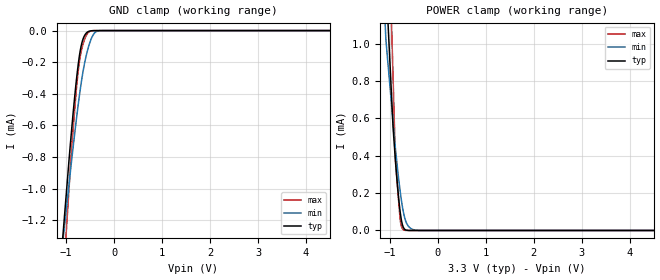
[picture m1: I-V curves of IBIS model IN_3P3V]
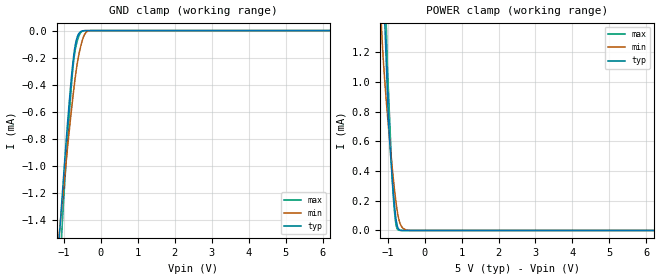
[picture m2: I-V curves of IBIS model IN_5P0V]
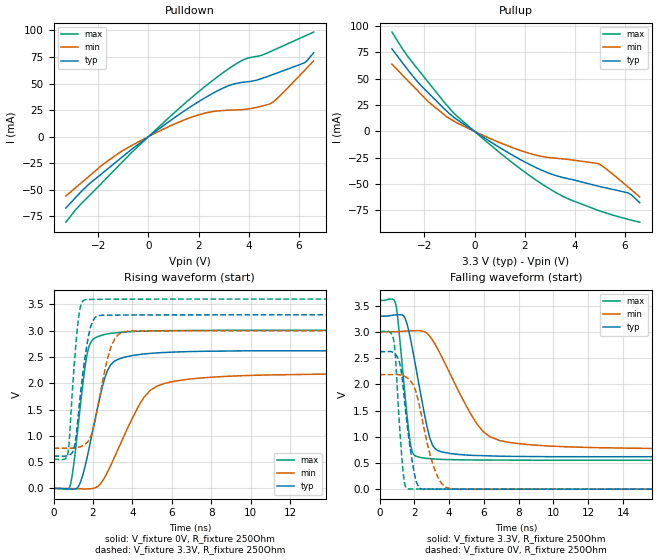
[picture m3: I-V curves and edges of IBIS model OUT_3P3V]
| Texas Instruments Incorporated
| Low-Power Single channel Digital Isolator
| Marketing part#   Voltage Range   Package-type   #pins/pkg drawing
| ISO7310C   3.0V - 5.5V   SOIC   8-pin D
[IBIS Ver]   4.1
[File name]   iso7310fc.ibs
[File Rev]   1.0
[Date]   09/30/2014
[Source]   Model built from spectre simulations at:
   Texas Instruments Incorporated.
   Analog-eLab, HPA
   12500 TI Blvd
   Dallas, TX -75243
   For Support e-mail: elab_ibis@list.ti.com
[Notes]   Revision History
   Rev 1.0: 09/30/2014
   - ccomp values are based on PVT settings:
   MIN: Low Voltage, High Temperature, Weak Process
   TYP: Nominal Voltage, Nominal Temperature, Nominal Process
   MAX: High Voltage, Low Temperature, Fast Process
   - C_comp although listed in numerical order of value are obtained from varying PVT conditions.
   For PVT conditions for each specific value, refer to the buffer description under respective [Model].
   IBIS model user is responsible for using appropriate C_comp to simulate for Signal Integrity.
[Disclaimer]  This model is designed as an aid for customers of Texas Instruments
 TI and its licensors and suppliers make no warranties, either expressed
 or implied, with respect to this  model, including the warranties of
 merchantability or fitness for a particular purpose.
 The model is provided solely on an "as is" basis. The entire risk as to
 its quality and performance is with the customer.
[Copyright] (C)Copyright 2014 Texas Instruments Incorporated.
   All rights reserved.
[Component]   ISO7310FCD
[Manufacturer]  Texas Instruments Incorporated
[Package]   |8-pin SOIC D package
|   typ   min   max
R_pkg   0.0731   0.0323   0.1488
L_pkg   2.0686n   1.4128n   3.1866n
C_pkg   0.4315p   0.3849p   0.5363p
[Pin]   signal_name   model_name   R_pin   L_pin   C_pin
1   VCC1   POWER   0.14877  3.18658n  0.42816p
2   IN   IN   0.09258  2.21690n  0.39598p
3   VCC1   POWER   0.08330  2.07043n  0.38782p
4   GND1   GND   0.05323  1.98056n  0.41432p
5   GND2   GND   0.05034  1.89272n  0.40532p
6   OUT   OUT   0.08318  2.07010n  0.38488p
7   GND2   GND   0.03229  1.41283n  0.49902p
8   VCC2   POWER   0.04142  1.71874n  0.53634p
[Model Selector] IN
IN_3P3V   3.3V Input
IN_5P0V   5.0V Input
[Model Selector] OUT
OUT_3P3V   3.3V Output
OUT_5P0V   5.0V Output
| Models and submodels in the file (4): IN_3P3V (Input), IN_5P0V (Input), OUT_3P3V (Output), OUT_5P0V (Output)
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|   IN_3P3V Model
[Model]   IN_3P3V
Model_type   Input
Vinl = 0.8
Vinh = 2
|   typ   min   max
|   (nom PVT)   (slow PVT)   (fast PVT)
C_comp   0.351pF   0.323pF   0.382pF
| Where   nom PVT is  Nominal Process, 3.3V, 27C
|   Fast PVT is Strong Process, 3.6V, -40C
|   Slow PVT is Weak Process, 3.0V, 150C
[Voltage Range]   3.3   3   3.6
[Temperature Range]   27   150   -40
[Power Clamp Reference]   3.3   3   3.6
[GND Clamp Reference]   0   0   0
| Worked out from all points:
|   GND clamp passes 1 mA (typ) near -0.99 V on its own axis
|   POWER clamp passes 1 mA (typ) near -1.02 V on its own axis
[GND Clamp]
|   Voltage   I(typ)   I(min)   I(max)
-3.3V     -10.39mA   -8.115mA   -12.82mA
-1.082V   -1.354mA   -1.374mA   -1.677mA
-933.9mV  -797.4uA   -956.1uA   -972uA
-884.4mV  -624.8uA   -817.9uA   -737uA
-785.4mV  -312.4uA   -559.5uA   -368.1uA
-735.9mV  -187.2uA   -440.5uA   -225.5uA
-696.3mV  -112uA     -353.2uA   -148.2uA
-646.8mV  -53.31uA   -257.7uA   -85.46uA
-528mV    -5.031uA   -97.34uA   -9.656uA
-419.1mV  -267.9nA   -19.35uA   -326.7nA
-260.7mV  0A         -360nA     0A
6.6V      0A         0A         0A
[POWER Clamp]
|   Voltage   I(typ)   I(min)   I(max)
-3.3V     19.39mA    14.36mA    23.85mA
-1.132V   1.605mA    1.287mA    2.629mA
-1.082V   1.342mA    1.019mA    2.178mA
-933.9mV  554.7uA    582.1uA    822.8uA
-884.4mV  378uA      439.9uA    371.2uA
-834.9mV  221.9uA    318uA      214.3uA
-785.4mV  99.44uA    209.9uA    57.41uA
-745.8mV  38.13uA    138uA      13.04uA
-706.2mV  10.91uA    83.53uA    2.199uA
-607.2mV  297.1nA    20.73uA    21.59nA
-419.1mV  0A         493.2nA    0A
6.6V      0A         0A         0A
|   IN_5P0V Model
[Model]   IN_5P0V
Model_type   Input
Vinl = 0.8
Vinh = 2
|   typ   min   max
|   (nom PVT)   (slow PVT)   (fast PVT)
C_comp   0.354pF   0.325pF   0.383pF
| Where   nom PVT is  Nominal Process, 5.0V, 27C
|   Fast PVT is Strong Process, 5.5V, -40C
|   Slow PVT is Weak Process, 4.5V, 150C
[Voltage Range]   5   4.5   5.5
[Temperature Range]   27   150   -40
[Power Clamp Reference]   5   4.5   5.5
[GND Clamp Reference]   0   0   0
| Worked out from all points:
|   GND clamp passes 1 mA (typ) near -0.99 V on its own axis
|   POWER clamp passes 1 mA (typ) near -1.02 V on its own axis
[GND Clamp]
|   Voltage   I(typ)   I(min)   I(max)
-5V       -17.38mA   -13.33mA   -21.61mA
-1.115V   -1.488mA   -1.468mA   -1.779mA
-1.055V   -1.255mA   -1.295mA   -1.484mA
-1.01V    -1.081mA   -1.167mA   -1.262mA
-875mV    -592.5uA   -792.6uA   -699.4uA
-755mV    -232uA     -485.3uA   -275uA
-710mV    -135.1uA   -382.4uA   -171.3uA
-650mV    -56.09uA   -263.4uA   -88.85uA
-515mV    -3.659uA   -84.59uA   -6.851uA
-410mV    -199.6nA   -16.03uA   -230.9nA
-290mV    0A         -798.1nA   0A
10V       0A         0A         0A
[POWER Clamp]
|   Voltage   I(typ)   I(min)   I(max)
-5V       33.77mA    25.3mA     41.21mA
-1.34V    3.142mA    2.182mA    4.333mA
-1.13V    1.742mA    1.192mA    2.29mA
-1.07V    1.343mA    978.4uA    1.706mA
-1.04V    1.143mA    881.8uA    1.414mA
-980mV    743.1uA    701.8uA    947uA
-875mV    346.2uA    416.8uA    332.1uA
-785mV    98.85uA    210uA      56.71uA
-710mV    12.46uA    88.64uA    2.617uA
-605mV    271.7nA    20.55uA    16.4nA
-425mV    0A         597.4nA    0A
10V       0A         0A         0A
|   Model OUT_3P3V
[Model]   OUT_3P3V
Model_type   Output
Polarity   Non-Inverting
Vmeas = 1.65
Vref = 3.3
Cref = 15pF
Rref = 250
|   typ   min   max
|   (fast PVT)   (slow PVT)   (nom PVT)
C_comp   0.728p   0.678p   0.736p
|C_comp (ON state)   0.797p   0.677p   0.792p
|C_comp (OFF state)   0.728p   0.678p   0.736p
| Where   nom PVT is  Nominal Process, 3.3V, 27C
|   Fast PVT is Strong Process, 3.6V, -40C
|   Slow PVT is Weak Process, 3.0V, 150C
[Voltage Range]   3.3   3   3.6
[Temperature Range]   27   150   -40
[Pullup Reference]   3.3   3   3.6
[Pulldown Reference]   0   0   0
[Power Clamp Reference]   3.3   3   3.6
[GND Clamp Reference]   0   0   0
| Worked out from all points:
|   slope of the pulldown table from 0 to 0.495 V, typ, clamps not added: 57 ohm
|   slope of the pullup table from 0 to 0.495 V, typ, clamps not added: 64.2 ohm
|   falling waveform, V_fixture 3.3V, R_fixture 250Ohm: 20-80 % time 916ps typ, 2.14ns min, 533ps max; typ from 3.3 V to 0.619 V
|   rising waveform, V_fixture 0V, R_fixture 250Ohm: 20-80 % time 931ps typ, 1.72ns min, 562ps max; typ from 0 V to 2.62 V
|   rising waveform, V_fixture 3.3V, R_fixture 250Ohm: 20-80 % time 518ps typ, 737ps min, 353ps max; typ from 0.615 V to 3.3 V
|   falling waveform, V_fixture 0V, R_fixture 250Ohm: 20-80 % time 578ps typ, 919ps min, 346ps max; typ from 2.62 V to 0 V
[Pulldown]
|   Voltage   I(typ)   I(min)   I(max)
-3.3V     -67.22mA   -55.92mA   -80.59mA
-2.389V   -44.97mA   -37.58mA   -56.09mA
-1.825V   -34.09mA   -26.21mA   -42.69mA
-696.3mV  -12.36mA   -8.646mA   -15.48mA
1.264V    21.55mA    14.15mA    27.39mA
2.65V     41.81mA    23.88mA    54.48mA
3.204V    47.99mA    24.92mA    63.99mA
3.729V    51.07mA    25.44mA    71.61mA
4.333V    53.29mA    27.64mA    75.66mA
4.897V    57.9mA     31.35mA    80.38mA
6.224V    69.48mA    62.11mA    94.52mA
6.6V      79.07mA    71.42mA    98.5mA
[Pullup]
|   Voltage   I(typ)   I(min)   I(max)
-3.3V     78.34mA    63.86mA    94.3mA
-2.686V   59.07mA    48.62mA    71.72mA
-2.32V    48.24mA    39.71mA    60.7mA
-1.825V   36.03mA    27.72mA    45.95mA
-1.099V   18.97mA    13.68mA    24.69mA
-696.3mV  11.13mA    8.021mA    14.38mA
1.68V     -24.78mA   -16.86mA   -32.82mA
2.511V    -35.01mA   -22.84mA   -47.11mA
3.343V    -42.61mA   -25.69mA   -59.28mA
4.947V    -52.03mA   -30.8mA    -75.05mA
6.125V    -58.4mA    -52.6mA    -83.42mA
6.6V      -67.78mA   -62.18mA   -86.22mA
[Ramp]
R_load = 250
|   typ   min   max
dV/dt_r   1.57011/9.31334e-10   1.30951/1.7182e-09   1.80445/5.62179e-10
dV/dt_f   1.60858/9.15648e-10   1.33827/2.13619e-09   1.8288/5.32895e-10
[Falling Waveform]
V_fixture = 3.3V
V_fixture_min = 3V
V_fixture_max = 3.6V
R_fixture = 250Ohm
C_fixture = 0F
|   Time   V(typ)   V(min)   V(max)
0s        3.3V       3V         3.6V
926.7ps   3.323V     3.003V     3.535V
1.391ns   3.302V     3.013V     2.046V
1.701ns   2.986V     3.018V     1.037V
2.122ns   2.256V     3.023V     625.9mV
2.72ns    1.202V     2.975V     586.9mV
3.195ns   771.1mV    2.761V     573.9mV
5.606ns   641.9mV    1.24V      556.8mV
6.908ns   629.1mV    927.6mV    554.9mV
19.9ns    619mV      769.6mV    552mV
[Rising Waveform]
V_fixture = 0V
V_fixture_min = 0V
V_fixture_max = 0V
R_fixture = 250Ohm
C_fixture = 0F
|   Time   V(typ)   V(min)   V(max)
0s        649.2pV    4.074nV    572.1pV
854.3ps   -10.96mV   -1.995mV   72.08mV
1.281ns   49.65mV    -6.905mV   1.3V
1.701ns   588.6mV    -8.959mV   2.553V
2.217ns   1.514V     31.88mV    2.883V
2.72ns    2.232V     302.2mV    2.936V
3.041ns   2.406V     554.2mV    2.954V
4.589ns   2.556V     1.736V     2.99V
5.606ns   2.584V     1.995V     2.999V
19.9ns    2.617V     2.183V     3.007V
[Rising Waveform]
V_fixture = 3.3V
V_fixture_min = 3V
V_fixture_max = 3.6V
R_fixture = 250Ohm
C_fixture = 0F
|   Time   V(typ)   V(min)   V(max)
0s        614.5mV    765mV      551.6mV
743.1ps   625.3mV    764.6mV    691.4mV
1.08ns    826mV      770.3mV    2.499V
1.218ns   1.252V     778.5mV    3.081V
1.571ns   2.429V     832.8mV    3.584V
1.876ns   3.071V     985.5mV    3.592V
2.107ns   3.25V      1.285V     3.594V
2.927ns   3.294V     2.707V     3.597V
3.58ns    3.296V     2.978V     3.598V
19.9ns    3.3V       3V         3.6V
[Falling Waveform]
|Gnd
V_fixture = 0V
V_fixture_min = 0V
V_fixture_max = 0V
R_fixture = 250Ohm
C_fixture = 0F
|   Time   V(typ)   V(min)   V(max)
0s        2.622V     2.184V     3.008V
815.5ps   2.601V     2.185V     2.839V
1.291ns   2.129V     2.171V     554.4mV
1.447ns   1.65V      2.152V     98.37mV
1.571ns   1.269V     2.127V     11.61mV
1.98ns    330.9mV    1.954V     2.742mV
2.22ns    54.41mV    1.701V     2.389mV
3.1ns     2.141mV    439.6mV    1.097mV
3.799ns   1.619mV    39.07mV    784.2uV
19.9ns    121uV      48.77uV    33.25uV
